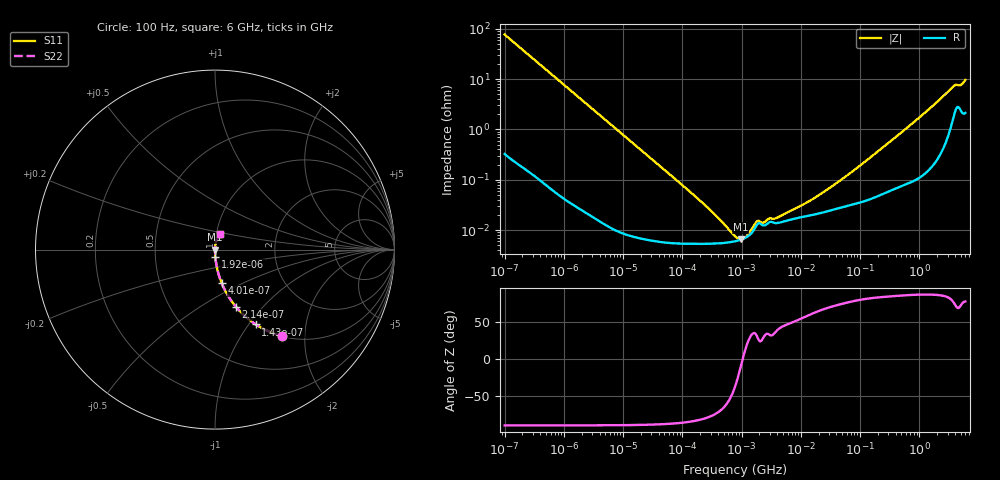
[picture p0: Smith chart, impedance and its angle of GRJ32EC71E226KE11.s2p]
!Murata Part Number: GRJ32EC71E226KE11
!These Parameters are Measured in Series Mode Connection
!Data Generated on Jun 19, 2026
!  o--ll--o
!Port1  Port2
!  o------o
!Operation Temp=25[degC], DC Bias Voltage=0[V]
!Freq. Start=100[Hz] Stop=6[GHz] 401[Steps]
# Hz S RI R 50
!Freq.(Hz) S11(Real) S11(Imag) S21(Real) S21(Imag) S12(Real) S12(Imag) S22(Real) S22(Imag)
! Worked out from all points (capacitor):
!   401 points, 100 Hz to 6 GHz, reference 50 ohm
!   read as one part in series: C = 20.6 uF near 109 Hz
!   lowest |Z| = 6.54 mohm at 969 kHz (marker M1)
!   series resonance near 1.047 MHz, so ESL is about 1.1 nH
!   S11 on the Smith chart (normalised r, x): 100 Hz: 1.01, -1.55; 143 Hz: 1.00, -1.08; 214 Hz: 1.00, -0.72; 401 Hz: 1.00, -0.39; 1.92 kHz: 1.00, -0.08; 6 GHz: 1.04, +0.19
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100  0.3745 -0.4819  0.6255 0.4819  0.6255 0.4819  0.3745 -0.4819
143  0.2272 -0.4169  0.7728 0.4169  0.7728 0.4169  0.2272 -0.4169
214  0.1168 -0.3189  0.8832 0.3189  0.8832 0.3189  0.1168 -0.3189
401  0.037 -0.1863  0.963 0.1863  0.963 0.1863  0.037 -0.1863
1920  0.0019 -0.0405  0.9981 0.0405  0.9981 0.0405  0.0019 -0.0405
2008  0.00175 -0.0387  0.9982 0.0387  0.9982 0.0387  0.00175 -0.0387
40335  6.22e-05 -0.00195  0.9999 0.00195  0.9999 0.00195  6.22e-05 -0.00195
231233  5.33e-05 -0.000324  0.9999 0.000324  0.9999 0.000324  5.33e-05 -0.000324
592111  5.67e-05 -9.08e-05  0.9999 9.08e-05  0.9999 9.08e-05  5.67e-05 -9.08e-05
774597  5.98e-05 -4.64e-05  0.9999 4.64e-05  0.9999 4.64e-05  5.98e-05 -4.64e-05
968953  6.43e-05 -1.18e-05  0.9999 1.18e-05  0.9999 1.18e-05  6.43e-05 -1.18e-05
1386327  8.1e-05 4.47e-05  0.9999 -4.47e-05  0.9999 -4.47e-05  8.1e-05 4.47e-05
1813585  0.000128 7.6e-05  0.9999 -7.6e-05  0.9999 -7.6e-05  0.000128 7.6e-05
2372521  0.000123 6.99e-05  0.9999 -6.99e-05  0.9999 -6.99e-05  0.000123 6.99e-05
3882480  0.000138 0.000106  0.9999 -0.000106  0.9999 -0.000106  0.000138 0.000106
1.555665e7  0.0002 0.000355  0.9998 -0.000355  0.9998 -0.000355  0.0002 0.000355
5.960426e7  0.000302 0.00117  0.9997 -0.00117  0.9997 -0.00117  0.000302 0.00117
3.124326e8  0.000623 0.00554  0.9994 -0.00554  0.9994 -0.00554  0.000623 0.00554
1.369159e9  0.00201 0.0236  0.998 -0.0236  0.998 -0.0236  0.00201 0.0236
3.666503e9  0.0195 0.0666  0.9805 -0.0666  0.9805 -0.0666  0.0195 0.0666
5.016141e9  0.0281 0.0689  0.9719 -0.0689  0.9719 -0.0689  0.0281 0.0689
6e9  0.0292 0.0896  0.9708 -0.0896  0.9708 -0.0896  0.0292 0.0896
